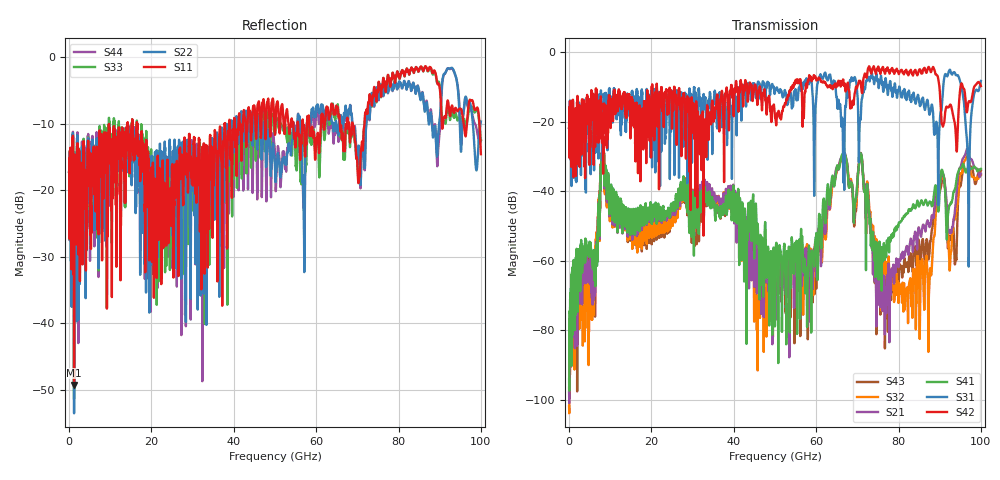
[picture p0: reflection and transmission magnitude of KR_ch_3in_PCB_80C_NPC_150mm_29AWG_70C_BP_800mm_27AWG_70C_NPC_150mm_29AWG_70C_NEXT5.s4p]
# GHz S RI R 45
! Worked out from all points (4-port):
!   4000 points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, 25 MHz to 100 GHz, reference 45 ohm
!   strongest paths, dB at 25 MHz, 25.02 GHz, 50.02 GHz, 75.03 GHz, 100 GHz:
!     S42: -21.8, -20.6, -18.8, -4.2, -9.7
!     S31: -21.8, -12.0, -11.4, -8.1, -8.3
!     S41: -94.0, -44.5, -71.8, -58.5, -33.6
!     S21: -97.8, -45.7, -66.1, -62.1, -35.0
!     S32: -101.9, -49.0, -70.4, -57.4, -35.3
!     S43: -96.5, -48.9, -71.1, -62.1, -34.1
!   lowest |S11| = -49.2 dB at 1.225 GHz (marker M1), VSWR 1.01, Z = 45.3 - j0.0216 ohm
!   |S11| at or under -10 dB: start of sweep to 14.15 GHz; 16.58 GHz to 37.77 GHz (21.2 GHz wide, 78 % of centre); 68.84 GHz to 71.74 GHz (2.901 GHz wide, 4.13 % of centre)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
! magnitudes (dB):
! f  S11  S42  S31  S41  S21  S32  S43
! 25 MHz  -17.2  -21.8  -21.8  -94.0  -97.8  -101.9  -96.5
! 1.225 GHz  -49.2  -27.8  -27.2  -66.5  -71.7  -83.8  -70.7
! 8.1 GHz  -17.5  -18.8  -22.7  -29.9  -30.3  -30.4  -30.1
! 46.08 GHz  -6.7  -11.0  -8.8  -56.0  -56.5  -64.5  -68.4
! 70.78 GHz  -15.0  -8.4  -19.5  -29.1  -30.0  -29.6  -29.1
! 76.58 GHz  -4.1  -5.2  -9.0  -58.8  -67.7  -60.7  -64.7
! 100 GHz  -14.6  -9.7  -8.3  -33.6  -35.0  -35.3  -34.1
